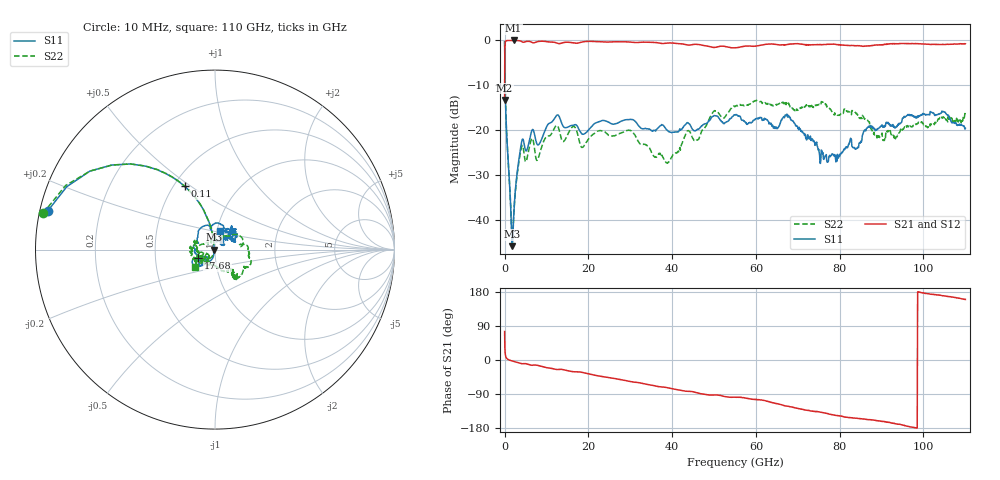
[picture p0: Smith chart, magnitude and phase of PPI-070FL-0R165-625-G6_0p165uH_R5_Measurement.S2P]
! Data measured by Modelithics Inc.  support@modelithics.com  813-866-6335  Tampa FL USA June 2025
! PPI-070FL-0R165-625-G6 _0p165uH measured on 5-mil thick RO3003G2 board, mounted in 2-port shunt configuration on a 50-ohm transmission line
# GHz S RI R 50.0
!freq ReS11 ImS11 ReS21 ImS21 ReS12 ImS12 ReS22 ImS22
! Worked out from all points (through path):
!   1207 points, 10 MHz to 110 GHz, reference 50 ohm
!   highest |S21| = -0.07 dB at 2.145 GHz (marker M1); lowest = -13.3 dB at 10 MHz (marker M2)
!   group delay of S21, straight-line fit = 5.09 ps
!   lowest |S11| = -45.7 dB at 1.853 GHz (marker M3), VSWR 1.01, Z = 49.5 - j0.0287 ohm
!   |S11| at or under -10 dB: 141.6 MHz to end of sweep
!   |S22| runs from -44.6 to -0.2 dB; largest |S21 - S12| = 0.078
!   S11 on the Smith chart (normalised r, x): 10 MHz: 0.02, +0.12; 110 MHz: 0.57, +0.47; 17.68 GHz: 0.83, -0.08; 110 GHz: 1.03, +0.21
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0.01  -0.9301 0.2178  0.0559 0.2101  0.0559 0.2101  -0.9584 0.2017
0.11  -0.1696 0.3532  0.8304 0.3504  0.8304 0.3504  -0.1697 0.3541
0.2  -0.0645 0.2218  0.9356 0.2163  0.9355 0.2163  -0.0641 0.2223
1.367977  -0.00549 0.0167  0.9916 -0.0185  0.9916 -0.0182  -0.00553 0.0171
1.853421  -0.00516 -0.00029  0.9909 -0.0472  0.991 -0.0467  -0.00586 0.000422
2.144687  -0.00536 -0.00882  0.9902 -0.0625  0.9902 -0.0626  -0.00662 -0.00782
4.183552  -0.0416 -0.0658  0.9458 -0.1636  0.946 -0.1628  -0.0475 -0.048
7.970015  -0.0533 -0.0435  0.9345 -0.2408  0.9345 -0.2408  -0.0336 -0.0341
12.53319  -0.1187 -0.0874  0.8381 -0.3935  0.838 -0.394  -0.0928 -0.0642
17.67889  -0.092 -0.0475  0.7956 -0.4838  0.7953 -0.4844  -0.0799 -0.0147
18.35852  -0.0781 -0.0489  0.8032 -0.5074  0.8033 -0.5075  -0.0602 -0.0241
29.7179  -0.1023 -0.0824  0.53 -0.7937  0.5325 -0.7924  -0.0998 -0.000805
36.7083  -0.1043 -0.0253  0.3165 -0.8768  0.3133 -0.878  -0.0372 0.038
39.03843  -0.0979 -0.00733  0.263 -0.8911  0.2673 -0.8899  -0.0208 0.0389
43.69869  -0.1195 0.0209  0.1138 -0.875  0.1112 -0.8753  0.0287 0.0944
55.05808  0.0103 0.1472  -0.1204 -0.8153  -0.1139 -0.8164  0.1845 0.00217
67.3  0.1004 0.1048  -0.4669 -0.759  -0.4282 -0.7858  0.1231 -0.1606
73.4  0.0458 0.0653  -0.6292 -0.6256  -0.5873 -0.6591  0.1053 -0.1489
79.5  0.013 0.0523  -0.7417 -0.4941  -0.7103 -0.5342  0.0969 -0.1102
91.7  0.1108 0.0433  -0.87 -0.2468  -0.8717 -0.2465  -0.0667 -0.0734
104.7  0.1151 0.1138  -0.8789 0.1604  -0.8832 0.1492  -0.1407 0.0129
110  0.0264 0.1018  -0.8545 0.3159  -0.8627 0.3014  -0.1099 -0.0971
